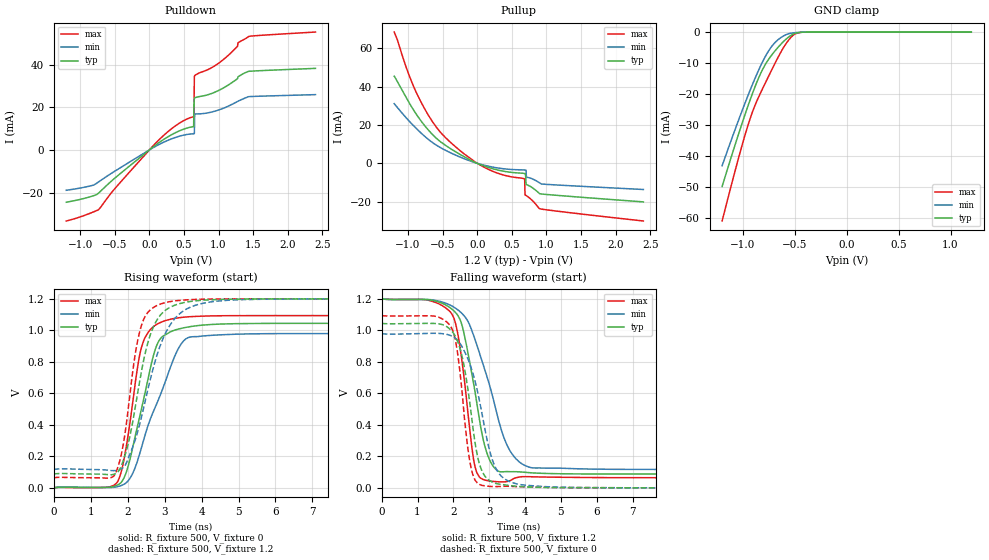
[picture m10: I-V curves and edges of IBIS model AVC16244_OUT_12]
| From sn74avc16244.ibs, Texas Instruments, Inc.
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[Model]   AVC16244_OUT_12
Model_type  3-state
Enable   Active-Low
Vref =   0
Rref =   2k
Cref =   15p
Vmeas =   0.6
| variable   typ   min   max
C_comp   3.96pF   3.32pF   4.86pF
| C_pullup   2.84pF   0.14pF   6.88pF
| C_pulldown   4.80pF   1.12pF   13.01pF
| C_tri-state   3.96pF   3.32pF   4.86pF
[Temperature Range]   40   100   -40
| Ambient temperature   25   85   -40
[Voltage range]   1.2   1.2   1.2
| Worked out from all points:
|   slope of the pulldown table from 0 to 0.18 V, typ, clamps not added: 41.3 ohm
|   slope of the pullup table from 0 to 0.18 V, typ, clamps not added: 75.9 ohm
|   GND clamp passes 1 mA (typ) near -0.53 V on its own axis
|   rising waveform, R_fixture 500, V_fixture 0: 20-80 % time 602ps typ, 888ps min, 426ps max; typ from 0 V to 1.04 V
|   falling waveform, R_fixture 500, V_fixture 1.2: 20-80 % time 532ps typ, 848ps min, 371ps max; typ from 1.2 V to 0.087 V
|   rising waveform, R_fixture 500, V_fixture 1.2: 20-80 % time 578ps typ, 785ps min, 415ps max; typ from 0.087 V to 1.2 V
|   falling waveform, R_fixture 500, V_fixture 0: 20-80 % time 425ps typ, 598ps min, 320ps max; typ from 1.04 V to 0 V
[GND Clamp]
| AVC16244_OUT_12
|   Voltage   I(typ)   I(min)   I(max)
-1.2V     -49.81mA   -43.12mA   -60.93mA
-1.065V   -35.33mA   -30.53mA   -43.53mA
-970mV    -25.69mA   -22.11mA   -32.16mA
-905mV    -19.57mA   -16.69mA   -25.52mA
-830mV    -13.44mA   -10.97mA   -19.64mA
-755mV    -8.942mA   -6.236mA   -14.44mA
-685mV    -5.853mA   -3.204mA   -9.722mA
-590mV    -2.479mA   -943.4uA   -4.03mA
-510mV    -576.6uA   -250.3uA   -914.9uA
-455mV    -143.1uA   -102.7uA   -185.2uA
-385mV    -21.43uA   -27.98uA   -14.82uA
1.2V      904pA      3.994nA    28.85pA
[Pulldown]
| AVC16244_OUT_12
|   Voltage   I(typ)   I(min)   I(max)
-1.2V     -24.58mA   -18.95mA   -33.4mA
-735mV    -20.3mA    -15.06mA   -28.1mA
140mV     3.462mA    2.573mA    4.781mA
640mV     10.98mA    7.608mA    15.63mA
645mV     21.39mA    7.616mA    15.69mA
650mV     24.35mA    7.636mA    34.23mA
655mV     24.51mA    16.53mA    34.97mA
660mV     24.57mA    16.86mA    35.1mA
1V        27.94mA    18.77mA    40.73mA
1.28V     34.34mA    22.9mA     50.3mA
1.445V    36.98mA    25.07mA    53.42mA
2.4V      38.34mA    26mA       55.42mA
[Pullup]
| AVC16244_OUT_12
|   Voltage   I(typ)   I(min)   I(max)
-1.2V     45.51mA    31.17mA    68.58mA
-950mV    29.56mA    20.73mA    42.76mA
-735mV    18.6mA     13.35mA    26.89mA
-520mV    10.96mA    7.962mA    15.74mA
-175mV    3.153mA    2.205mA    4.538mA
230mV     -2.893mA   -2.023mA   -4.269mA
685mV     -5.328mA   -3.511mA   -8.179mA
690mV     -5.367mA   -3.522mA   -16.51mA
705mV     -11.02mA   -3.556mA   -16.81mA
710mV     -11.09mA   -7.24mA    -16.92mA
900mV     -15.81mA   -10.2mA    -23.72mA
2.4V      -20.15mA   -13.67mA   -30.14mA
[Ramp]
| AVC16244_OUT_12
| variable   typ   min   max
dV/dt_r   0.63/6.08E-10   0.59/8.89E-10   0.66/4.34E-10
dV/dt_f   0.67/5.37E-10   0.65/8.51E-10   0.70/3.81E-10
R_load = 500
[Rising Waveform]
| AVC16244_OUT_12
R_fixture =   500
C_fixture =   0
L_fixture =   0
V_fixture =   0
V_fixture_min = 0
V_fixture_max = 0
|   Time   V(typ)   V(min)   V(max)
0s        18.81nV    103.6nV    513.5pV
1.635ns   9.619mV    3.778mV    17.77mV
1.82ns    33.4mV     14.42mV    97.6mV
2.01ns    135.9mV    44.17mV    332.9mV
2.305ns   432mV      201.8mV    820.2mV
2.47ns    604mV      334.8mV    954.6mV
2.865ns   940.9mV    579.4mV    1.048V
3.35ns    1.007V     874.9mV    1.079V
3.66ns    1.022V     955.5mV    1.086V
70ns      1.044V     979.3mV    1.094V
[Falling Waveform]
| AVC16244_OUT_12
R_fixture =   500
C_fixture =   0
L_fixture =   0
V_fixture =   1.2
V_fixture_min = 1.2
V_fixture_max = 1.2
|   Time   V(typ)   V(min)   V(max)
0s        1.2V       1.2V       1.2V
1.27ns    1.196V     1.195V     1.193V
1.95ns    1.136V     1.156V     1.106V
2.175ns   1.073V     1.121V     907.6mV
2.615ns   593.7mV    934.1mV    124.8mV
2.875ns   267.5mV    750.5mV    49.91mV
3.165ns   122mV      516.1mV    39.85mV
3.615ns   102.6mV    222.6mV    49.77mV
4.28ns    94.1mV     125.9mV    69.76mV
70ns      87.35mV    116.2mV    63.9mV
[Rising Waveform]
| AVC16244_OUT_12
R_fixture =   500
C_fixture =   0
L_fixture =   0
V_fixture =   1.2
V_fixture_min = 1.2
V_fixture_max = 1.2
|   Time   V(typ)   V(min)   V(max)
0s        87.35mV    116.2mV    63.9mV
1.595ns   84.36mV    109.3mV    70.57mV
1.915ns   197.8mV    137.2mV    326.1mV
2.215ns   527.4mV    313.6mV    865.8mV
2.445ns   824.8mV    522mV      1.076V
2.68ns    1.013V     750.5mV    1.143V
2.96ns    1.115V     949.9mV    1.173V
3.545ns   1.177V     1.129V     1.193V
6.485ns   1.2V       1.199V     1.2V
70ns      1.2V       1.2V       1.2V
[Falling Waveform]
| AVC16244_OUT_12
R_fixture =   500
C_fixture =   0
L_fixture =   0
V_fixture =   0
V_fixture_min = 0
V_fixture_max = 0
|   Time   V(typ)   V(min)   V(max)
0s        1.044V     979.3mV    1.094V
1.92ns    1.004V     967.3mV    1.027V
2.075ns   952.2mV    945.6mV    914.4mV
2.235ns   841.8mV    898.4mV    623.7mV
2.52ns    427.9mV    745.4mV    102mV
2.73ns    149.8mV    550.1mV    21.43mV
3.055ns   40.34mV    200.7mV    8.656mV
3.625ns   13.33mV    34.89mV    9.276mV
5.4ns     663.8uV    2.341mV    1.538mV
70ns      25.22nV    130.1nV    8.638nV
